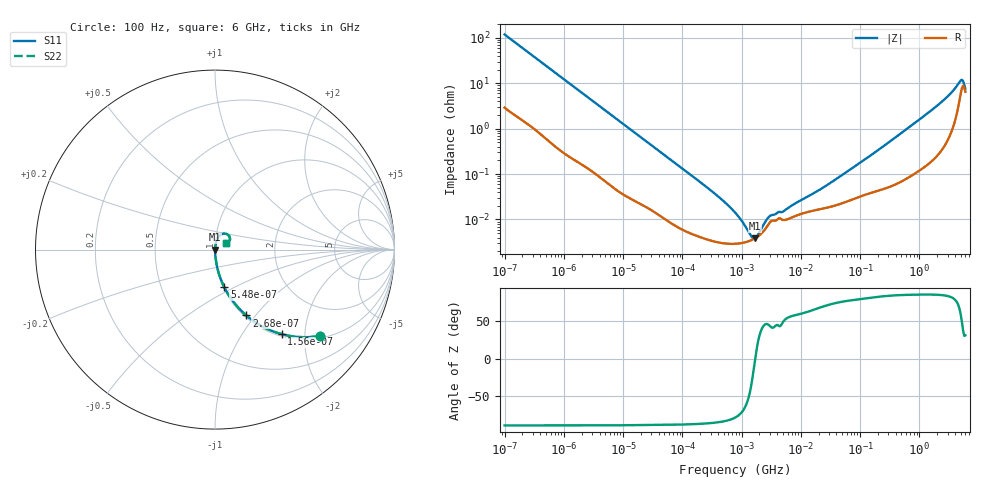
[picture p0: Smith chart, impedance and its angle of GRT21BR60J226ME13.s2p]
!Murata Part Number: GRT21BR60J226ME13
!These Parameters are Measured in Series Mode Connection
!Data Generated on Jun 19, 2026
!  o--ll--o
!Port1  Port2
!  o------o
!Operation Temp=25[degC], DC Bias Voltage=0[V]
!Freq. Start=100[Hz] Stop=6[GHz] 401[Steps]
# Hz S RI R 50
!Freq.(Hz) S11(Real) S11(Imag) S21(Real) S21(Imag) S12(Real) S12(Imag) S22(Real) S22(Imag)
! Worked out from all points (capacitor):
!   401 points, 100 Hz to 6 GHz, reference 50 ohm
!   read as one part in series: C = 13.4 uF near 109 Hz
!   lowest |Z| = 3.83 mohm at 1.658 MHz (marker M1)
!   series resonance near 1.697 MHz, so ESL is about 660 pH
!   S11 on the Smith chart (normalised r, x): 100 Hz: 1.06, -2.37; 156 Hz: 1.04, -1.52; 268 Hz: 1.02, -0.90; 548 Hz: 1.01, -0.44; 6 GHz: 1.13, +0.08
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100  0.5826 -0.4811  0.4174 0.4811  0.4174 0.4811  0.5826 -0.4811
156  0.3709 -0.4708  0.6291 0.4708  0.6291 0.4708  0.3709 -0.4708
268  0.1745 -0.3669  0.8255 0.3669  0.8255 0.3669  0.1745 -0.3669
548  0.0518 -0.2097  0.9482 0.2097  0.9482 0.2097  0.0518 -0.2097
981  0.0182 -0.1225  0.9818 0.1225  0.9818 0.1225  0.0182 -0.1225
2008  0.0054 -0.0613  0.9946 0.0613  0.9946 0.0613  0.0054 -0.0613
40335  0.000135 -0.00325  0.9999 0.00325  0.9999 0.00325  0.000135 -0.00325
330837  3.34e-05 -0.000396  1 0.000396  1 0.000396  3.34e-05 -0.000396
774597  2.91e-05 -0.00014  1 0.00014  1 0.00014  2.91e-05 -0.00014
1013323  3.04e-05 -8.71e-05  1 8.71e-05  1 8.71e-05  3.04e-05 -8.71e-05
1658239  3.81e-05 -3.7e-06  1 3.7e-06  1 3.7e-06  3.81e-05 -3.7e-06
2594782  6.53e-05 6.89e-05  0.9999 -6.89e-05  0.9999 -6.89e-05  6.53e-05 6.89e-05
3245845  9.35e-05 8.31e-05  0.9999 -8.31e-05  0.9999 -8.31e-05  9.35e-05 8.31e-05
5079039  9.73e-05 0.000116  0.9999 -0.000116  0.9999 -0.000116  9.73e-05 0.000116
1.555665e7  0.000155 0.000328  0.9998 -0.000328  0.9998 -0.000328  0.000155 0.000328
4.165952e7  0.000211 0.000786  0.9998 -0.000786  0.9998 -0.000786  0.000211 0.000786
3.124326e8  0.000545 0.00509  0.9995 -0.00509  0.9995 -0.00509  0.000545 0.00509
2.142435e9  0.00396 0.0342  0.996 -0.0342  0.996 -0.0342  0.00396 0.0342
3.352442e9  0.0108 0.0575  0.9892 -0.0575  0.9892 -0.0575  0.0108 0.0575
4.796499e9  0.0502 0.0896  0.9498 -0.0896  0.9498 -0.0896  0.0502 0.0896
5.245841e9  0.079 0.0766  0.921 -0.0766  0.921 -0.0766  0.079 0.0766
6e9  0.0623 0.0349  0.9377 -0.0349  0.9377 -0.0349  0.0623 0.0349
